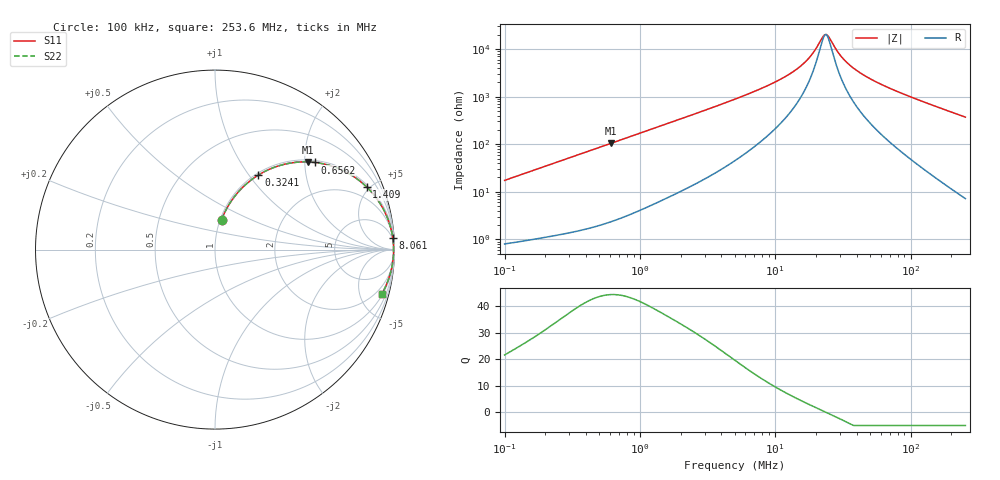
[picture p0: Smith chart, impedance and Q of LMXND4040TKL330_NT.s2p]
! LMXND4040TKL330_NT  S-PARAMETER MODEL  ( Standard Model )
! Model Generated by TAIYO YUDEN Corporation (https://www.yuden.co.jp/en/)
! Version 1.0
! TAIYO YUDEN Control No. 20251120
! Copyright(c) 2025 TAIYO YUDEN CO.,LTD. All Rights Reserved.
! Product Description (link to TY-COMPAS)
! https://ds.yuden.co.jp/TYCOMPAS/or/detail?pn=LMXND4040TKL330MNT&u=M
! Products Name : Inductors
! Characteristics :
!  Inductance : 33 [uH] , SRF(min) : 12 [MHz] , DC Resistance(max) : 0.552 [Ohm]
!  Rated Current : Saturation  700 [mA] , Temp Rise  880 [mA] (40 [degC])
!  Case Size : 4.0 x 4.0 / 0.157 x 0.157 [mm/inch] , Thickness : 1.8 / 0.071 [mm/inch]
!  (Conditions: Temperature = 25 [degC] , DC Bias Current = 0 [A])
! External Node Assignments :
!  1  o---GGG---o  2
! GND o---------o GND
! Frequency Range : 0.1MHz  -  253.640152MHz  [ 402 STEP ]
# MHz S RI R 50
! Freq[MHz].  S11 Real  S11 Imag  S21 Real  S21 Imag  S12 Real  S12 Imag  S22 Real  S22 Imag
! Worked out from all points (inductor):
!   401 points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, 100 kHz to 253.6 MHz, reference 50 ohm
!   read as one part in series: L = 27.6 uH near 104 kHz
!   highest Q = 44.4 at 606.7 kHz (marker M1), where L = 27.2 uH
!   self-resonance near 23.22 MHz
!   S11 on the Smith chart (normalised r, x): 100 kHz: 1.02, +0.35; 324.1 kHz: 1.03, +1.11; 656.2 kHz: 1.05, +2.24; 1.409 MHz: 1.13, +4.79; 8.061 MHz: 3, +30; 253.6 MHz: 1.14, -7.41
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0.1  0.0366 0.1661  0.9634 -0.1661  0.9634 -0.1661  0.0366 0.1661
0.190918  0.1055 0.2912  0.8945 -0.2912  0.8945 -0.2912  0.1055 0.2912
0.324065  0.2417 0.4154  0.7583 -0.4154  0.7583 -0.4154  0.2417 0.4154
0.371712  0.2932 0.4431  0.7068 -0.4431  0.7068 -0.4431  0.2932 0.4431
0.606695  0.5175 0.4886  0.4825 -0.4886  0.4825 -0.4886  0.5175 0.4886
0.656164  0.5554 0.4858  0.4446 -0.4858  0.4446 -0.4858  0.5554 0.4858
1.381698  0.8403 0.3534  0.1597 -0.3534  0.1597 -0.3534  0.8403 0.3534
1.409041  0.8453 0.3487  0.1547 -0.3487  0.1547 -0.3487  0.8453 0.3487
2.43904  0.9387 0.224  0.0613 -0.224  0.0613 -0.224  0.9387 0.224
5.03627  0.9819 0.1102  0.0181 -0.1102  0.0181 -0.1102  0.9819 0.1102
8.060502  0.9906 0.0644  0.00942 -0.0644  0.00942 -0.0644  0.9906 0.0644
13.68191  0.9942 0.0286  0.00583 -0.0286  0.00583 -0.0286  0.9942 0.0286
16.32081  0.9947 0.0189  0.00533 -0.0189  0.00533 -0.0189  0.9947 0.0189
18.72042  0.9949 0.0117  0.00508 -0.0117  0.00508 -0.0117  0.9949 0.0117
22.33112  0.9951 0.00274  0.00494 -0.00274  0.00494 -0.00274  0.9951 0.00274
23.2237  0.9951 0.000775  0.00493 -0.000775  0.00493 -0.000775  0.9951 0.000775
24.15197  0.9951 -0.00119  0.00492 0.00119  0.00492 0.00119  0.9951 -0.00119
29.96185  0.9949 -0.0121  0.00506 0.0121  0.00506 0.0121  0.9949 -0.0121
35.74074  0.9946 -0.0214  0.00537 0.0214  0.00537 0.0214  0.9946 -0.0214
47.02309  0.9937 -0.0373  0.0063 0.0373  0.0063 0.0373  0.9937 -0.0373
69.58603  0.9908 -0.0652  0.00919 0.0652  0.00919 0.0652  0.9908 -0.0652
253.6402  0.9279 -0.2491  0.0721 0.2491  0.0721 0.2491  0.9279 -0.2491
